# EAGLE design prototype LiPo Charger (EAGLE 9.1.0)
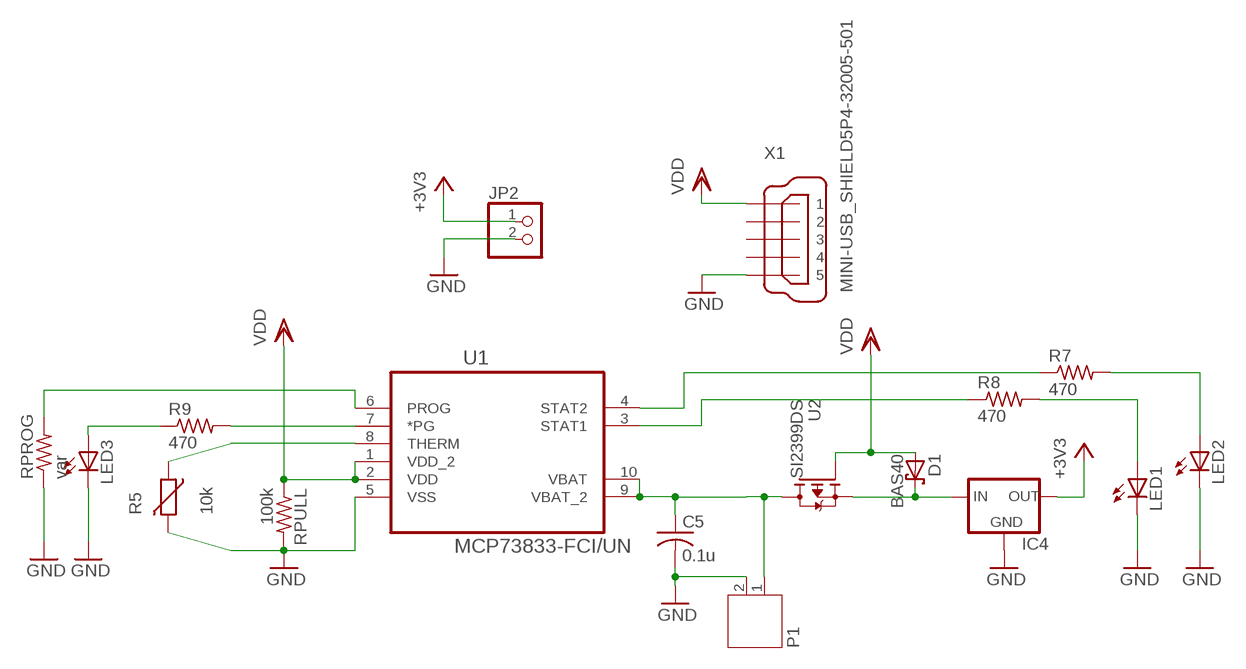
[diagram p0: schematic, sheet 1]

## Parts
C5  0.1u  C-USC0603  [C0603]
D1  BAS40  [SOT23]
IC4  XC63FPM  [SOT23]
JP2  PINHD-1X2  [1X02]
LED1  LEDCHIPLED_0603  [CHIPLED_0603]
LED2  LEDCHIPLED_0603  [CHIPLED_0603]
LED3  LEDCHIPLED_0603  [CHIPLED_0603]
P1  JST-PH2  [JST-PH2]
R5  10k  VARISTORCN0805  [CT/CN0805]
R7  470  R-US_R0603  [R0603]
R8  470  R-US_R0603  [R0603]
R9  470  R-US_R0603  [R0603]
RPROG  var  R-US_R0603  [R0603]
RPULL  100k  R-US_R0603  [R0603]
U1  MCP73833-FCI/UN  [SOP50P490X110-10N]
U2  SI2399DS  [SOT23]
X1  MINI-USB_SHIELD5P4-32005-501  [32005-501]

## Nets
+3V3: IC4.2(OUT) JP2.1
GND: C5.2 IC4.1(GND) JP2.2 LED1.C LED2.C LED3.C P1.2 R5.2 RPROG.1 RPULL.2 U1.5(VSS) X1.5
N$1: C5.1 P1.1 U1.9(VBAT_2) U1.10(VBAT) U2.3(D)
N$2: LED1.A R8.2
N$3: LED2.A R7.2
N$4: R5.1 U1.8(THERM)
N$5: RPROG.2 U1.6(PROG)
N$6: LED3.A R9.1
N$8: R8.1 U1.3(STAT1)
N$9: R7.1 U1.4(STAT2)
N$10: R9.2 U1.7(*PG)
N$12: D1.3(C) IC4.3(IN) U2.2(S)
VDD: D1.1(A) RPULL.1 U1.1(VDD_2) U1.2(VDD) U2.1(G) X1.1
Unconnected: X1.2 X1.3 X1.4 X1.M1(S1) X1.M2(S2) X1.M3(S3) X1.M4(S4)

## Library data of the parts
C5 = resistor:C-US: CAPACITOR, American symbol
D1 = diode:BAS40: Silicon Schottky Diodes
IC4 = v-reg:XC63FP: Positiv Voltage Regulators www.torex.co.jp/english/product/pro02/pdf/0201_xc62fp.pdf
JP2 = pinhead:PINHD-1X2: PIN HEADER
LED1-LED3 = led:LED: LED
P1 = jst-ph:JST-PH2
R5 = varistor:VARISTOR: VARISTOR
R7-R9 RPROG RPULL = resistor:R-US_: RESISTOR, American symbol
U1 = MCP73833:MCP73833-FCI/UN: LI-ION/LI-POLY CONTROLLERS; MPN: MCP73833-FCI/UN; OC_FARNELL: 1605576; OC_NEWARK: 88K5666; PACKAGE: MSOP10; SUPPLIER: Microchip
U2 = Custom:SI2399DS
X1 = con-cypressindustries:MINI-USB_SHIELD5P4-: MINI USB-B R/A W/O POST 5 pol. Source: www.cypressindustries.com; OC_FARNELL: unknown; OC_NEWARK: unknown

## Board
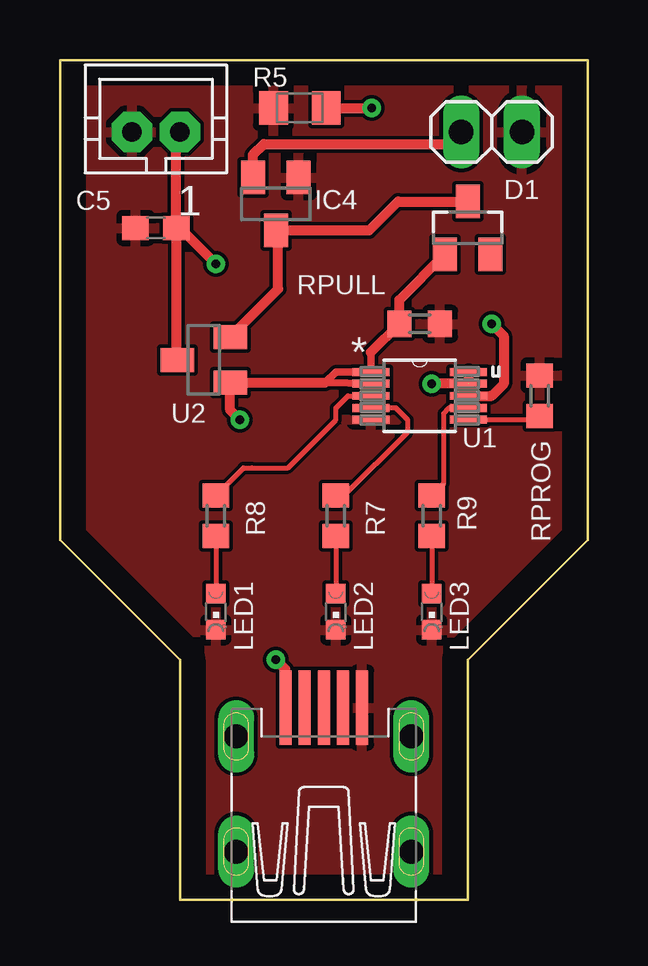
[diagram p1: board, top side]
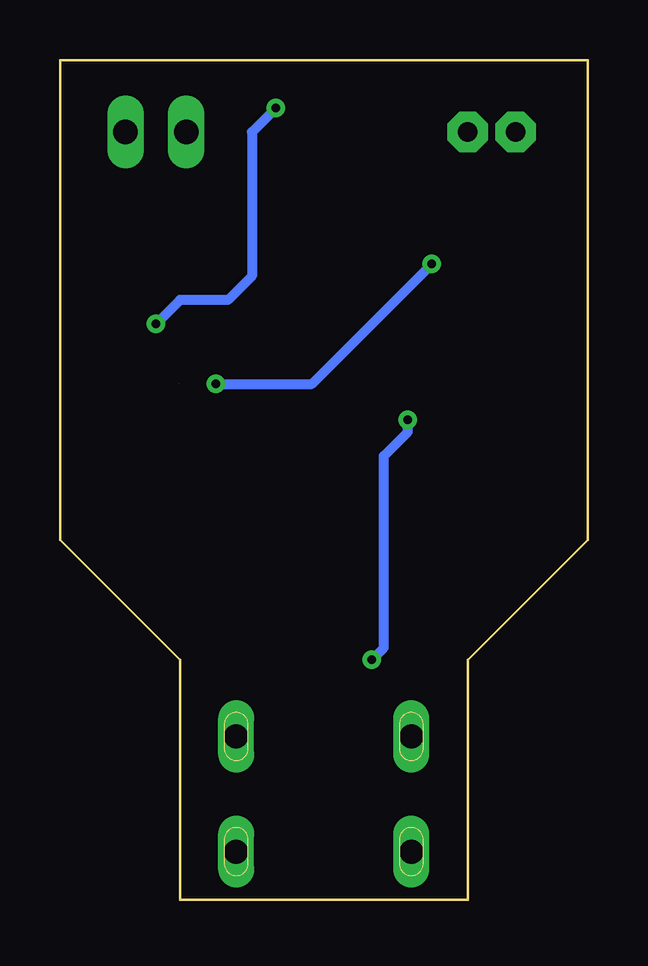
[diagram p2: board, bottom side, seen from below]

Size 22 x 35 mm. Coordinates in mm from the lower left corner, seen from the top.
Outline: 5,0 17,0 17,10 22,15 22,35 0,35 0,15 5,10 5,0
Copper layers (1*16): Top 0.035mm / dielectric 1.5mm / Bottom 0.035mm
Design rules "default": minimum track width 6mil, minimum drill 0.35mm, track to track 6mil, track to pad 6mil, pad to pad 6mil, via to via 6mil, smd to smd 6mil, copper to edge 40mil, drill to drill 6mil, minimum pad ring 10mil, minimum via ring 8mil, stop-mask expansion 4mil, vias tented up to drill 0mil, thermal gap 10mil

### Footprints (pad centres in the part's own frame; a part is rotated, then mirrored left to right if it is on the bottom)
C0603 = smd 1.1 x 1: 1 -0.85,0; 2 0.85,0
SOT23 = smd 1 x 1.4: 1 -0.95,-1.1; 2 0.95,-1.1; 3 0,1.1
1X02 = drill 1.016 long: 1 -1.27,0; 2 1.27,0
CHIPLED_0603 = smd 0.8 x 0.8: A 0,-0.75; C 0,0.75
JST-PH2 = drill 0.813 pad 1.676 octagon: 1 1,0; 2 -1,0
CT/CN0805 = smd 1.2 x 1.4: 1 -1.1,0; 2 1.1,0
R0603 = smd 1 x 1.1: 1 -0.85,0; 2 0.85,0
SOP50P490X110-10N = smd 1.524 x 0.33: 1 -2.032,0.991; 2 -2.032,0.508; 3 -2.032,0; 4 -2.032,-0.508; 5 -2.032,-0.991; 6 2.032,-0.991; 7 2.032,-0.508; 8 2.032,0; 9 2.032,0.508; 10 2.032,0.991
32005-501 = smd 3.1 x 0.5: 1 3,1.6; 2 3,0.8; 3 3,0; 4 3,-0.8; 5 3,-1.6 | drill 1 pad 1.422 long: M1 -3,3.65; M2 -3,-3.65; M3 1.8,3.65; M4 1.8,-3.65

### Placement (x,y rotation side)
C5  4,28 180 top
D1  17,28 0 top
IC4  9,29 180 top
JP2  18,32 0 top
LED1  6.5,12 180 top
LED2  11.5,12 180 top
LED3  15.5,12 180 top
P1  4,32 0 top
R5  10,33 180 top
R7  11.5,16 270 top
R8  6.5,16 270 top
R9  15.5,16 90 top
RPROG  20,21 270 top
RPULL  15,24 0 top
U1  15,21 0 top
U2  6,22.5 90 top
X1  11,5 90 top

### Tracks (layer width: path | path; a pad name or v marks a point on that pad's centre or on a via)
+3V3
  Top 0.406: IC4.2 8.05,31.05 8.5,31.5 16.23,31.5 JP2.1
GND
  pour Top: 0,35 22,35 22,15 17,10 17,0 5,0 5,10 0,15
N$1  (via drill 0.35)  (1 unrouted)
  Top 0.406: C5.1 5,27.85 5.15,27.85 v6.5,26.5 | C5.1 4.85,31.85 P1.1 | U1.10 17.03,21.52 15.52,21.52 v15.5,21.5 | C5.1 4.85,22.55 U2.3
  Bottom 0.406: v15.5,21.5 11.5,21.5 v6.5,26.5
N$2
  Top 0.203: R8.2 LED1.A
N$3
  Top 0.203: R7.2 LED2.A
N$4  (via drill 0.35)
  Top 0.406: R5.1 v13,33 | v18,24 18.5,23.5 18.5,21.5 18,21 | 18,21 17.95,21 | 17.95,21 18,21 | 18,21 17.95,21 | U1.8 17.95,21
  Bottom 0.406: v13,33 14,32 14,26 15,25 17,25 v18,24
N$5
  Top 0.203: U1.6 19.86,20.01 RPROG.2
N$6
  Top 0.203: R9.1 LED3.A
N$8
  Top 0.203: R8.1 7.65,18 8,18 9.5,18 11.5,20 11.5,20.5 12,21 U1.3
N$9
  Top 0.203: U1.4 13.99,20.49 14,20.5 14.5,20 14.5,19.5 11.85,16.85 R7.1
N$10
  Top 0.203: R9.2 16,17.35 16,20.26 16.23,20.49 U1.7
N$12
  Top 0.406: D1.3 14.1,29.1 12.9,27.9 IC4.3 9.1,27.8 9.1,25.45 U2.2
VDD  (via drill 0.35)
  Top 0.305: U1.2 11.05,21.55 11.51,21.99 U1.1 12.97,22.82
  Top 0.406: X1.1 9.4,9.6 v9,10 | 12.97,22.82 RPULL.1 14.15,25 D1.1 | v7.5,20 7.1,20.4 U2.1 11.05,21.55
  Bottom 0.406: v9,10 8.5,10.5 8.5,18.5 7.5,19.5 v7.5,20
